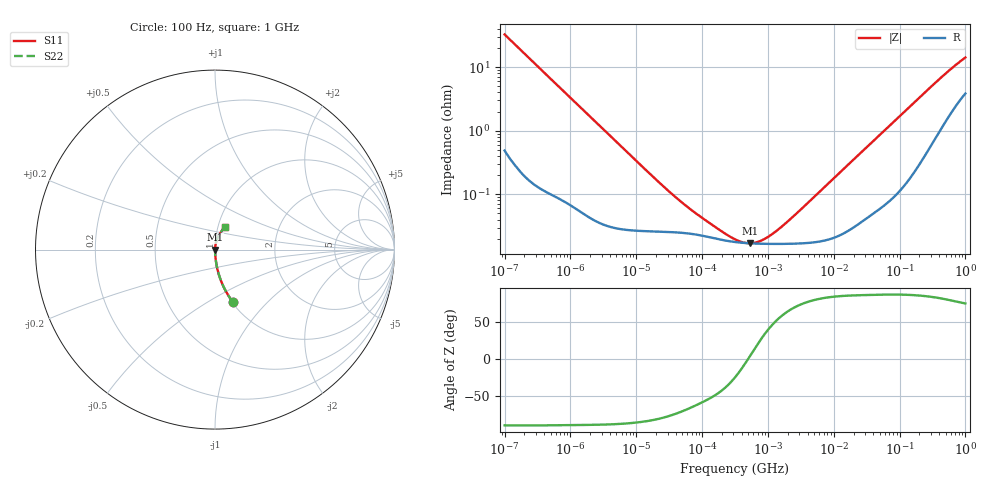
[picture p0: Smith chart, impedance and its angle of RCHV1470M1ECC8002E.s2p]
! RCHV1470M1ECC8002E  S-PARAMETER MODEL  (AEC-Q200 qualified)
! Model Generated by ELNA Corporation (http://www.ty-top.com)
! Version 1.0
! ELNA Control No.240229
! Copyright (c) 2024 ELNA CO.,LTD. All Rights Reserved.
! Products Name : CONDUCTIVE POLYMER HYBRID ALUMINUM ELECTROLYTIC CAPACITORS
! Characteristics :
!  Capacitance  :  47uF  ,  Rated voltage  :  16V
!  Operating Temp. Range  :  -55 to +105 degC  ,  Endurance  :  10000hr at 105 degC
!  Dimension D  :  5mm  ,  Dimension L  :  5.8mm
! Frequency Range : 100Hz - 1GHz
! External Node Assignments :
!  1  o---| |---o  2
# MHz S RI R 50
!Freq[MHz].  S11 Real  S11 Imag  S21 Real  S21 Imag  S12 Real  S12 Imag  S22 Real  S22 Imag
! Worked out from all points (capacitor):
!   401 points, 100 Hz to 1 GHz, reference 50 ohm
!   read as one part in series: C = 48.7 uF near 108 Hz
!   lowest |Z| = 17 mohm at 533.9 kHz (marker M1)
!   series resonance near 501.3 kHz, so ESL is about 2.1 nH
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0.0001  0.1002 -0.2929  0.8998 0.2929  0.8998 0.2929  0.1002 -0.2929
0.000113  0.0806 -0.2654  0.9194 0.2654  0.9194 0.2654  0.0806 -0.2654
0.000162  0.0413 -0.1929  0.9587 0.1929  0.9587 0.1929  0.0413 -0.1929
0.000309  0.0124 -0.1046  0.9876 0.1046  0.9876 0.1046  0.0124 -0.1046
0.000613  0.00376 -0.0534  0.9962 0.0534  0.9962 0.0534  0.00376 -0.0534
0.001488  0.00101 -0.0223  0.999 0.0223  0.999 0.0223  0.00101 -0.0223
0.022131  0.000261 -0.00152  0.9997 0.00152  0.9997 0.00152  0.000261 -0.00152
0.04217  0.000251 -0.000814  0.9997 0.000814  0.9997 0.000814  0.000251 -0.000814
0.074131  0.000236 -0.000479  0.9998 0.000479  0.9998 0.000479  0.000236 -0.000479
0.194984  0.000193 -0.000181  0.9998 0.000181  0.9998 0.000181  0.000193 -0.000181
0.316228  0.000178 -8.25e-05  0.9998 8.25e-05  0.9998 8.25e-05  0.000178 -8.25e-05
0.419276  0.000172 -3.15e-05  0.9998 3.15e-05  0.9998 3.15e-05  0.000172 -3.15e-05
0.533949  0.000169 1.12e-05  0.9998 -1.12e-05  0.9998 -1.12e-05  0.000169 1.12e-05
0.767361  0.000167 7.82e-05  0.9998 -7.82e-05  0.9998 -7.82e-05  0.000167 7.82e-05
1.148154  0.000166 0.000166  0.9998 -0.000166  0.9998 -0.000166  0.000166 0.000166
1.938653  0.000166 0.000323  0.9998 -0.000323  0.9998 -0.000323  0.000166 0.000323
4.704354  0.000175 0.000831  0.9998 -0.000831  0.9998 -0.000831  0.000175 0.000831
69.9842  0.000916 0.0118  0.9991 -0.0118  0.9991 -0.0118  0.000916 0.0118
184.0772  0.00349 0.0303  0.9965 -0.0303  0.9965 -0.0303  0.00349 0.0303
412.0975  0.0141 0.0641  0.9859 -0.0641  0.9859 -0.0641  0.0141 0.0641
695.825  0.0328 0.0977  0.9672 -0.0977  0.9672 -0.0977  0.0328 0.0977
1000  0.0535 0.1246  0.9465 -0.1246  0.9465 -0.1246  0.0535 0.1246
